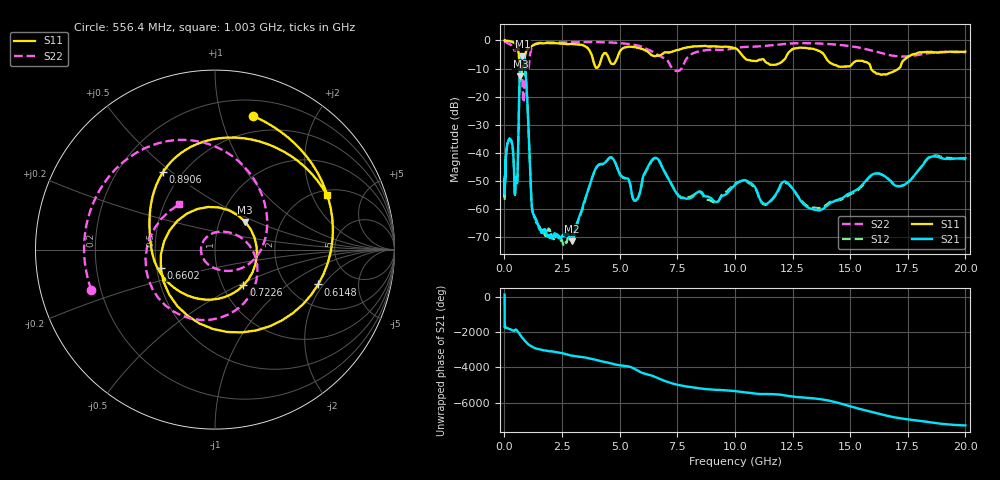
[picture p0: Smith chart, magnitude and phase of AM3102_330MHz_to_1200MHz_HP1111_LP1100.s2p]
! Date/Time: Tue, Sep 11, 2018 5:24 PM
! Network Analyzer: Agilent Technologies E8362B Rev: A.07.50.63
! Sweep from 0.010 to 20.000 GHz, 1601 Points, Sweep Type: LOG
! Power Supply: 4.949 V, 0.001 A
# Hz S DB R 50
!freq MagS11 AngS11 MagS21 AngS21 MagS12 AngS12 MagS22 AngS22
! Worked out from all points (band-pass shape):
!   1601 points, 10 MHz to 20 GHz, reference 50 ohm
!   highest |S21| = -5.58 dB at 779.7 MHz (marker M1); lowest = -71.5 dB at 2.92 GHz (marker M2)
!   |S21| within 3 dB of the highest: 693.3 MHz to 884.5 MHz (191.2 MHz wide, 24.2 % of centre)
!   lowest |S11| = -12.8 dB at 695.6 MHz (marker M3), VSWR 1.59, Z = 66.3 + j21.6 ohm
!   |S11| at or under -10 dB: 660.8 MHz to 768 MHz (107.2 MHz wide, 15 % of centre); 15.91 GHz to 17.11 GHz (1.202 GHz wide, 7.28 % of centre)
!   |S22| runs from -22.1 to -0.2 dB; largest |S21 - S12| = 0.0061
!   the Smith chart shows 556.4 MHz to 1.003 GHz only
!   S11 on the Smith chart (normalised r, x): 556.4 MHz: 0.34, +1.27; 614.8 MHz: 2.89, -1.78; 660.2 MHz: 0.53, -0.12; 722.6 MHz: 1.25, -0.53; 890.6 MHz: 0.39, +0.47; 1.003 GHz: 2.21, +2.60
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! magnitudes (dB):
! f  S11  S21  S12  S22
! 10 MHz  0.0  -52.3  -49.2  -0.2
! 35.55 MHz  -0.1  -46.3  -46.6  -0.5
! 126.4 MHz  -0.2  -37.0  -36.9  -0.9
! 334.7 MHz  -0.5  -36.7  -36.6  -2.1
! 447.2 MHz  -1.0  -54.1  -54.4  -3.6
! 556.4 MHz  -2.2  -50.6  -50.8  -2.8
! 614.8 MHz  -4.3  -29.6  -29.9  -2.9
! 660.2 MHz  -9.9  -14.0  -14.1  -4.4
! 695.6 MHz  -12.8  -8.4  -8.4  -6.7
! 722.6 MHz  -11.9  -6.6  -6.6  -8.7
! 779.7 MHz  -9.6  -5.6  -5.7  -14.7
! 890.6 MHz  -5.7  -9.0  -9.2  -12.0
! 1.003 GHz  -3.2  -22.9  -23.1  -9.9
! 1.201 GHz  -1.9  -59.6  -59.9  -2.3
! 1.59 GHz  -1.0  -68.3  -67.3  -0.9
! 2.92 GHz  -1.2  -71.5  -69.3  -0.7
! 4.092 GHz  -9.2  -44.4  -44.2  -0.6
! 5.652 GHz  -2.4  -57.0  -57.2  -1.6
! 6.549 GHz  -5.6  -41.8  -41.9  -4.6
! 7.771 GHz  -2.8  -56.1  -55.8  -8.6
! 13.61 GHz  -3.6  -60.5  -59.7  -1.1
! 20 GHz  -4.0  -41.9  -42.3  -4.2
